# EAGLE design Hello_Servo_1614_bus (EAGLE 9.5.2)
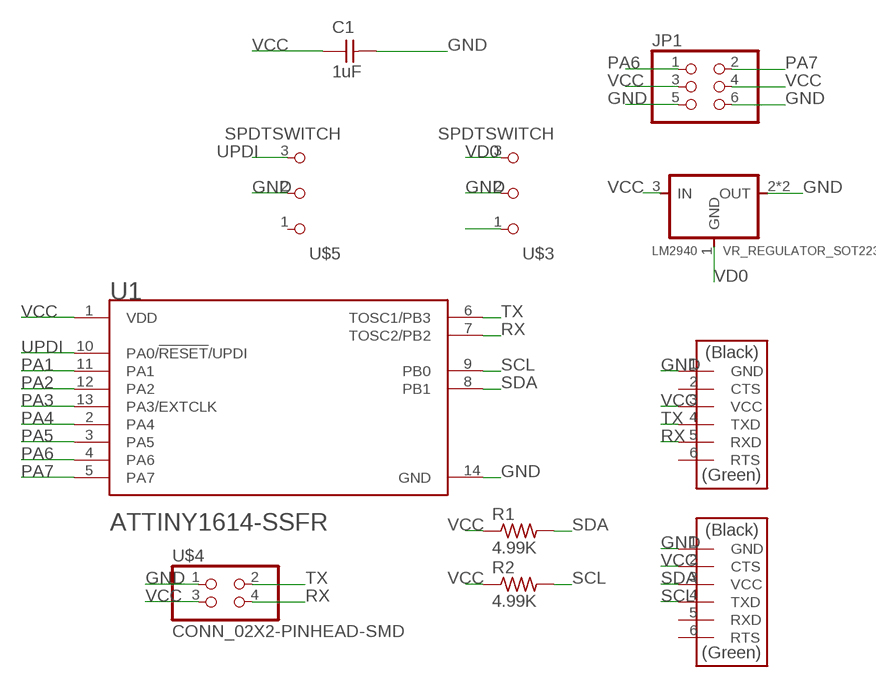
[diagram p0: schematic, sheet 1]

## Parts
C1  1uF  CAP_UNPOLARIZEDFAB  [C1206FAB]
JP1  CONN_03X2-PINHEAD-SMD  [2X03SMD]
LM2940  VR_REGULATOR_SOT223  [SOT223]
R1  4.99K  R1206FAB  [R1206FAB]
R2  4.99K  R1206FAB  [R1206FAB]
U1  MICROCHIP_ATTINY1614-SSFRMICROCHIP_ATTINY1614-SSFR_0_1  [MICROCHIP_ATTINY1614]
U$1  CONN_06_FTDI-SMD-HEADER  [1X06SMD]
U$2  CONN_06_FTDI-SMD-HEADER  [1X06SMD]
U$3  SPDTSWITCH  [SPDTSWITCH]
U$4  CONN_02X2-PINHEAD-SMD  [2X02SMD]
U$5  SPDTSWITCH  [SPDTSWITCH]

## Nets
GND: C1.2 JP1.5 JP1.6 LM2940.2(OUT) LM2940.4(OUT) U1.14(GND) U$1.1(GND) U$2.1(GND) U$3.2 U$4.1 U$5.2
N$2: U$3.1
PA1: U1.11(PA1)
PA2: U1.12(PA2)
PA3: U1.13(PA3/EXTCLK)
PA4: U1.2(PA4)
PA5: U1.3(PA5)
PA6: JP1.1 U1.4(PA6)
PA7: JP1.2 U1.5(PA7)
RX: U1.7(TOSC2/PB2) U$2.5(RXD) U$4.4
SCL: R2.2 U1.9(PB0) U$1.4(TXD)
SDA: R1.2 U1.8(PB1) U$1.3(VCC)
TX: U1.6(TOSC1/PB3) U$2.4(TXD) U$4.2
UPDI: U1.10(PA0/!RESET!/UPDI) U$5.3
VCC [New Class]: C1.1 JP1.3 JP1.4 LM2940.3(IN) R1.1 R2.1 U1.1(VDD) U$1.2(CTS) U$2.3(VCC) U$4.3
VD0: LM2940.1(GND) U$3.3
Unconnected: U$1.5(RXD) U$1.6(RTS) U$2.2(CTS) U$2.6(RTS) U$5.1

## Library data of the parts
C1 = fab:CAP_UNPOLARIZED
JP1 = fab:CONN_03X2-PINHEAD-SMD: PIN HEADER
LM2940 = fab:VR_REGULATOR_SOT223
R1 R2 = fab:R: Resistor (US Symbol)
U1 = Microchip - ATTINY1614-SSFR:MICROCHIP_ATTINY1614-SSFR: IC MCU 8BIT 16KB FLASH 14SOIC; AUTOMOTIVE: No; CENTROID_NOT_SPECIFIED: No; CORE_ARCHITECTURE: AVR; DATASHEET: http://ww1.microchip.com/downloads/en/DeviceDoc/ATtiny1614-DataSheet-DS40001995B.pdf; DATA_BUS_WIDTH: 8bits; DEVICE_CLASS_L1: Integrated Circuits (ICs); DEVICE_CLASS_L2: Embedded Processors and Controllers; DEVICE_CLASS_L3: Microcontrollers; DIGIKEY_DESCRIPTION: IC MCU 8BIT 16KB FLASH 14SOIC; DIGIKEY_PART_NUMBER: ATTINY1614-SSFRCT-ND; FOOTPRINT_PARAMETERS_1: {"fp_type":"SOIC_narrow","params":{"N":{"nom":14,"long name":"Number of leads","min":null,"max":null,"short name":"N","type":"count"},"A":{"nom":false,"long name":"Height","min":false,"max":1750000,"short name":"A","type":"measurement"},"A1":{"nom":false,"long name":"Package clearance","min":100000,"max":250000,"short name":"A1","type":"measurement"},"A2":{"nom":false,"long name":"Package height","min":1250000,"max":false,"short name":"A2","type":"measurement"},"D":{"nom":8650000,"long name":"Package length","min":8550000,"max":8750000,"short name":"D","type":"measurement"},"E":{"nom":6000000,"long name":"Width w/ leads","min":5800000,"max":6200000,"short name":"E","type":"measurement"},"E1":{"nom":3900000,"long name":"Package width","min":3800000,"max":4000000,"short name":"E1","type":"measurement"},"B":{"nom":false,"long name":"Lead width","min":310000,"max":510000,"short name":"B","type":"measurement"},"C":{"nom":false,"long name":"Lead thickness","min":100000,"max":250000,"short name":"C","type":"measurement"},"e":{"nom":1270000,"long name":"Lead pitch","min":null,"max":null,"short name":"e","type":"measurement"},"L":{"nom":false,"long name":"Lead foot length","min":400000,"max":1270000,"short name":"L","type":"measurement"},"PHI":{"nom":false,"long name":"Lead foot angle","min":0,"max":8000000,"short name":"PHI","type":"measurement"},"HT":{"default":"No","long name":"Thermal pad","type":"multichoiceparent","short name":"HT","children":[]},"offset x":{"nom":0,"long name":"X Center offset","min":null,"max":null,"short name":"offset x","type":"measurement"},"offset y":{"nom":0,"long name":"Y Center offset","min":null,"max":null,"short name":"offset y","type":"measurement"},"LS":{"default":"Rounded rectangle","long name":"Land shape","type":"multichoice","short name":"LS"},"LS1":{"default":"Rectangle","long name":"Land shape (Pin 1)","type":"multichoice","short name":"LS1"},"solder toe":{"nom":550000,"long name":"Solder fillet (toe)","min":null,"max":null,"short name":"solder toe","type":"fixedmeasurement"},"solder heel":{"nom":450000,"long name":"Solder fillet (heel)","min":null,"max":null,"short name":"solder heel","type":"fixedmeasurement"},"solder side":{"nom":50000,"long name":"Solder fillet (side)","min":null,"max":null,"short name":"solder side","type":"fixedmeasurement"},"courtyard":{"nom":500000,"long name":"Courtyard","min":null,"max":null,"short name":"courtyard","type":"fixedmeasurement"},"SF":{"default":"A","long name":"Packing level","type":"multichoiceparent","short name":"SF","help":"http://support.upverter.com/customer/portal/articles/978783-what-is-a-footprint-packing-level","children":["solder toe","solder heel","solder side","courtyard"]}}}; FOOTPRINT_PARAMETERS_2: {"fp_type":"SOIC_narrow","params":{"N":{"nom":14,"long name":"Number of leads","min":null,"max":null,"short name":"N","type":"count"},"A":{"nom":false,"long name":"Height","min":false,"max":1750000,"short name":"A","type":"measurement"},"A1":{"nom":false,"long name":"Package clearance","min":100000,"max":250000,"short name":"A1","type":"measurement"},"A2":{"nom":false,"long name":"Package height","min":1250000,"max":false,"short name":"A2","type":"measurement"},"D":{"nom":8650000,"long name":"Package length","min":8550000,"max":8750000,"short name":"D","type":"measurement"},"E":{"nom":6000000,"long name":"Width w/ leads","min":5800000,"max":6200000,"short name":"E","type":"measurement"},"E1":{"nom":3900000,"long name":"Package width","min":3800000,"max":4000000,"short name":"E1","type":"measurement"},"B":{"nom":false,"long name":"Lead width","min":310000,"max":510000,"short name":"B","type":"measurement"},"C":{"nom":false,"long name":"Lead thickness","min":100000,"max":250000,"short name":"C","type":"measurement"},"e":{"nom":1270000,"long name":"Lead pitch","min":null,"max":null,"short name":"e","type":"measurement"},"L":{"nom":false,"long name":"Lead foot length","min":400000,"max":1270000,"short name":"L","type":"measurement"},"PHI":{"nom":false,"long name":"Lead foot angle","min":0,"max":8000000,"short name":"PHI","type":"measurement"},"HT":{"default":"No","long name":"Thermal pad","type":"multichoiceparent","short name":"HT","children":[]},"offset x":{"nom":0,"long name":"X Center offset","min":null,"max":null,"short name":"offset x","type":"measurement"},"offset y":{"nom":0,"long name":"Y Center offset","min":null,"max":null,"short name":"offset y","type":"measurement"},"LS":{"default":"Rounded rectangle","long name":"Land shape","type":"multichoice","short name":"LS"},"LS1":{"default":"Rectangle","long name":"Land shape (Pin 1)","type":"multichoice","short name":"LS1"},"solder toe":{"nom":350000,"long name":"Solder fillet (toe)","min":null,"max":null,"short name":"solder toe","type":"fixedmeasurement"},"solder heel":{"nom":350000,"long name":"Solder fillet (heel)","min":null,"max":null,"short name":"solder heel","type":"fixedmeasurement"},"solder side":{"nom":30000,"long name":"Solder fillet (side)","min":null,"max":null,"short name":"solder side","type":"fixedmeasurement"},"courtyard":{"nom":250000,"long name":"Courtyard","min":null,"max":null,"short name":"courtyard","type":"fixedmeasurement"},"SF":{"default":"B","long name":"Packing level","type":"multichoiceparent","short name":"SF","help":"http://support.upverter.com/customer/portal/articles/978783-what-is-a-footprint-packing-level","children":["solder toe","solder heel","solder side","courtyard"]}}}; FOOTPRINT_PARAMETERS_3: {"fp_type":"SOIC_narrow","params":{"N":{"nom":14,"long name":"Number of leads","min":null,"max":null,"short name":"N","type":"count"},"A":{"nom":false,"long name":"Height","min":false,"max":1750000,"short name":"A","type":"measurement"},"A1":{"nom":false,"long name":"Package clearance","min":100000,"max":250000,"short name":"A1","type":"measurement"},"A2":{"nom":false,"long name":"Package height","min":1250000,"max":false,"short name":"A2","type":"measurement"},"D":{"nom":8650000,"long name":"Package length","min":8550000,"max":8750000,"short name":"D","type":"measurement"},"E":{"nom":6000000,"long name":"Width w/ leads","min":5800000,"max":6200000,"short name":"E","type":"measurement"},"E1":{"nom":3900000,"long name":"Package width","min":3800000,"max":4000000,"short name":"E1","type":"measurement"},"B":{"nom":false,"long name":"Lead width","min":310000,"max":510000,"short name":"B","type":"measurement"},"C":{"nom":false,"long name":"Lead thickness","min":100000,"max":250000,"short name":"C","type":"measurement"},"e":{"nom":1270000,"long name":"Lead pitch","min":null,"max":null,"short name":"e","type":"measurement"},"L":{"nom":false,"long name":"Lead foot length","min":400000,"max":1270000,"short name":"L","type":"measurement"},"PHI":{"nom":false,"long name":"Lead foot angle","min":0,"max":8000000,"short name":"PHI","type":"measurement"},"HT":{"default":"No","long name":"Thermal pad","type":"multichoiceparent","short name":"HT","children":[]},"offset x":{"nom":0,"long name":"X Center offset","min":null,"max":null,"short name":"offset x","type":"measurement"},"offset y":{"nom":0,"long name":"Y Center offset","min":null,"max":null,"short name":"offset y","type":"measurement"},"LS":{"default":"Rounded rectangle","long name":"Land shape","type":"multichoice","short name":"LS"},"LS1":{"default":"Rectangle","long name":"Land shape (Pin 1)","type":"multichoice","short name":"LS1"},"solder toe":{"nom":150000,"long name":"Solder fillet (toe)","min":null,"max":null,"short name":"solder toe","type":"fixedmeasurement"},"solder heel":{"nom":250000,"long name":"Solder fillet (heel)","min":null,"max":null,"short name":"solder heel","type":"fixedmeasurement"},"solder side":{"nom":10000,"long name":"Solder fillet (side)","min":null,"max":null,"short name":"solder side","type":"fixedmeasurement"},"courtyard":{"nom":100000,"long name":"Courtyard","min":null,"max":null,"short name":"courtyard","type":"fixedmeasurement"},"SF":{"default":"C","long name":"Packing level","type":"multichoiceparent","short name":"SF","help":"http://support.upverter.com/customer/portal/articles/978783-what-is-a-footprint-packing-level","children":["solder toe","solder heel","solder side","courtyard"]}}}; FOOTPRINT_VARIANT_NAME_0: Recommended_Land_Pattern; FOOTPRINT_VARIANT_NAME_1: IPC_A; FOOTPRINT_VARIANT_NAME_2: IPC_B; FOOTPRINT_VARIANT_NAME_3: IPC_C; FREQUENCY: 16MHz; HEIGHT: 1.75mm; INTERFACE: I2C,SPI,UART,USART,2-Wire,LIN,IrDA; IPC_LAND_PATTERN_NAME: SOIC127P600X175-14; LEAD_FREE: Yes; MAX_SUPPLY_VOLTAGE: 5.5V; MEMORY_SIZE: 16KBytes; MEMORY_TYPE: FLASH; MF: Microchip; MFG_PACKAGE_IDENT: C04-065-D3X; MFG_PACKAGE_IDENT_DATE: 0; MFG_PACKAGE_IDENT_REV: D; MIN_SUPPLY_VOLTAGE: 1.8V; MOUSER_DESCRIPTION: 8-Bit AVR Microcontroller 16Kbyte Flash 2Kbyte SRAM 14-Pin SOIC T/R; MOUSER_PART_NUMBER: 556-ATTINY1614SSFR; MPN: ATTINY1614-SSFR; NOMINAL_SUPPLY_CURRENT: 2.6-10200uA; NUMBER_OF_A/D_CONVERTERS: 2; NUMBER_OF_ADC_CHANNELS: 14; NUMBER_OF_CORES: 1; NUMBER_OF_I/OS: 12; NUMBER_OF_I2C_CHANNELS: 1; NUMBER_OF_PWM_CHANNELS: 1; NUMBER_OF_SPI_CHANNELS: 1; NUMBER_OF_TIMERS/COUNTERS: 5; NUMBER_OF_UART_CHANNELS: 1; PACKAGE: SOIC14; PREFIX: U; RAM_SIZE: 2KBytes; ROHS: Yes; STANDOFF_HEIGHT: 0.1mm; TEMPERATURE_RANGE_HIGH: +125°C; TEMPERATURE_RANGE_LOW: -40°C; VERIFICATION_VERSION: 0.0.0.3
U$1 U$2 = fab:CONN_06_FTDI-SMD-HEADER
U$3 U$5 = fab:SPDTSWITCH
U$4 = fab:CONN_02X2-PINHEAD-SMD

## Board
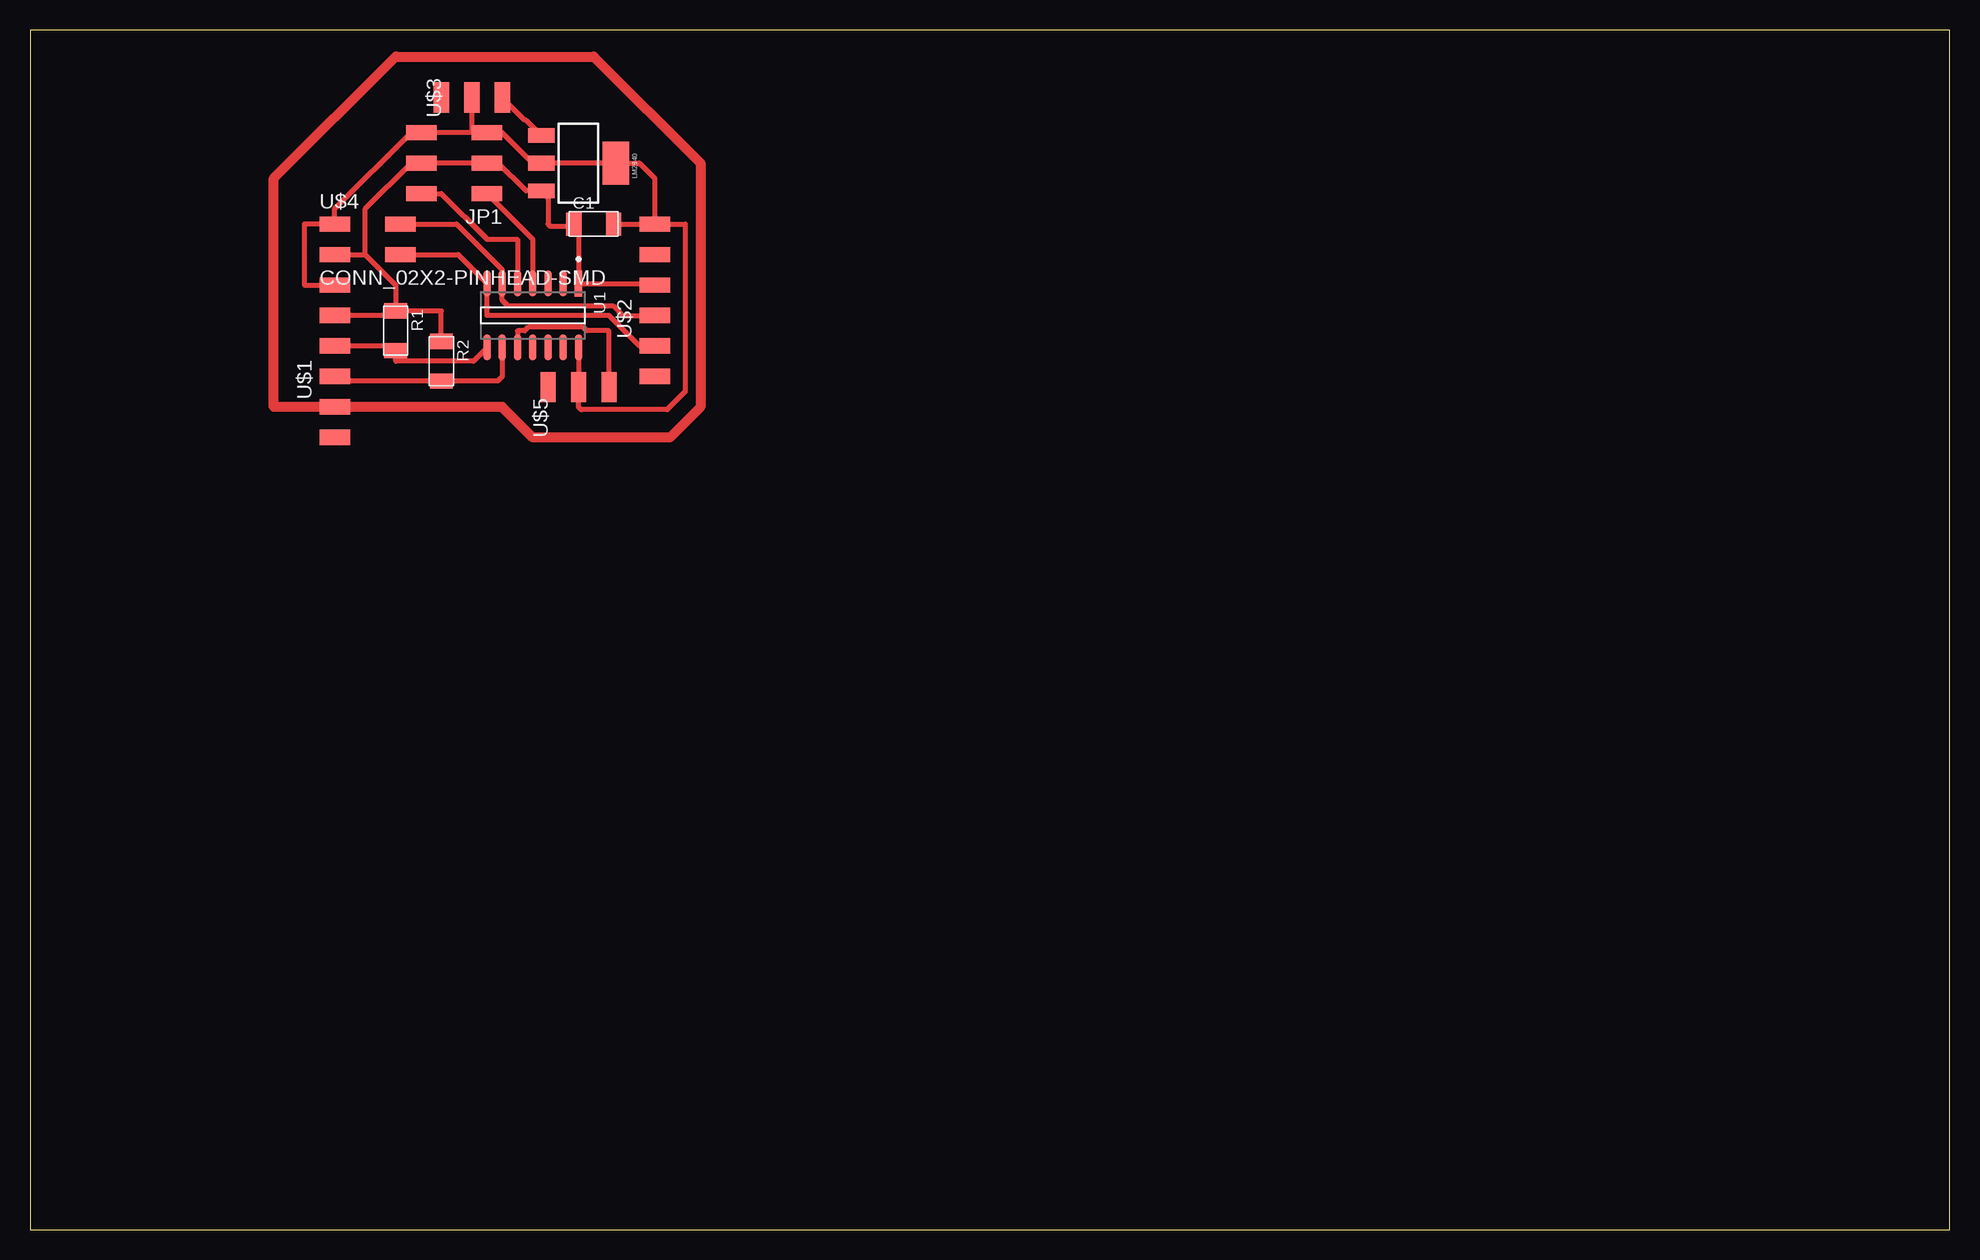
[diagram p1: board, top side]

Size 160 x 100 mm. Coordinates in mm from the lower left corner, seen from the top.
Outline: 0,0 160,0 160,100 0,100 0,0
Copper layers (1*16): Top 0.035mm / dielectric 1.5mm / Bottom 0.035mm
Design rules "default *": minimum track width 16mil, minimum drill 0.35mm, track to track 16mil, track to pad 16mil, pad to pad 16mil, via to via 16mil, smd to smd 6mil, copper to edge 40mil, drill to drill 6mil, minimum pad ring 10mil, minimum via ring 8mil, stop-mask expansion 4mil, vias tented up to drill 0mil, thermal gap 10mil

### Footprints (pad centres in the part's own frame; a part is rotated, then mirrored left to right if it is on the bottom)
C1206FAB = smd 1.27 x 1.905: 1 -1.651,0; 2 1.651,0
2X03SMD = smd 2.54 x 1.27: 1 -2.54,2.54; 2 2.92,2.54; 3 -2.54,0; 4 2.92,0; 5 -2.54,-2.54; 6 2.92,-2.54
SOT223 = smd 1.219 x 2.235: 1 -2.311,-3.099; 2 0,-3.099; 3 2.311,-3.099 | smd 3.6 x 2.2: 4 0,3.099
R1206FAB = smd 1.27 x 1.905: 1 -1.651,0; 2 1.651,0
MICROCHIP_ATTINY1614 = smd 2.169 x 0.622: 1 -2.67,3.81; 2 -2.67,2.54; 3 -2.67,1.27; 4 -2.67,0; 5 -2.67,-1.27; 6 -2.67,-2.54; 7 -2.67,-3.81; 8 2.67,-3.81; 9 2.67,-2.54; 10 2.67,-1.27; 11 2.67,0; 12 2.67,1.27; 13 2.67,2.54; 14 2.67,3.81
1X06SMD = smd 2.54 x 1.27: 1 0,6.35; 2 0,3.81; 3 0,1.27; 4 0,-1.27; 5 0,-3.81; 6 0,-6.35
SPDTSWITCH = smd 2.54 x 1.27: 1 0.38,2.54; 2 0.38,0; 3 0.38,-2.54
2X02SMD = smd 2.54 x 1.27: 1 -2.54,1.27; 2 2.92,1.27; 3 -2.54,-1.27; 4 2.92,-1.27

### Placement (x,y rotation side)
C1  46.99,83.82 0 top
JP1  35.56,88.9 180 top
LM2940  45.72,88.9 270 top
R1  30.48,74.93 270 top
R2  34.29,72.39 270 top
U1  41.91,76.2 270 top
U$1  25.4,72.39 0 top
U$2  52.07,77.47 0 top
U$3  36.83,93.98 90 top
U$4  27.94,82.55 0 top
U$5  45.72,69.85 90 top

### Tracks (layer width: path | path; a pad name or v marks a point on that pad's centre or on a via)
GND
  Top 0.406: C1.2 U$2.1 | U1.14 U$5.2 45.72,68.58 45.95,68.35 53.11,68.35 54.61,69.85 54.61,83.82 U$2.1 | U$3.2 36.83,91.44 JP1.5 | U$2.1 52.07,87.63 50.8,88.9 LM2940.4 LM2940.2 41.91,88.9 39.37,91.44 JP1.5 | JP1.5 JP1.6 31.75,91.44 25.4,85.09 U$4.1 22.86,83.82 22.86,78.74 U$1.1
N$1
  Top 0.813: 30.48,97.79 46.99,97.79 55.88,88.9 55.88,68.58 53.34,66.04 41.91,66.04 39.37,68.58 20.32,68.58 20.32,87.63 30.48,97.79
PA6
  Top 0.406: JP1.1 41.91,82.55 U1.4
PA7
  Top 0.406: JP1.2 34.29,86.36 38.1,82.55 40.64,82.55 U1.5
RX
  Top 0.406: U$2.5 50.8,73.66 48.26,76.2 38.1,76.2 U1.7 35.69,81.28 U$4.4
SCL
  Top 0.406: U1.9 39.37,71.12 38.99,70.74 R2.2 25.78,70.74 U$1.4
SDA
  Top 0.406: U1.8 36.96,72.39 30.48,72.39 R1.2 30.1,73.66 U$1.3
TX
  Top 0.406: U$2.4 49.41,76.2 48.6,77.01 39.83,77.01 39.37,77.47 39.37,78.74 U1.6 39.37,80.01 35.56,83.82 U$4.2
UPDI
  Top 0.406: U$5.3 48.26,74.93 46.4,74.93 46.1,75.22 41.53,75.22 41.23,74.93 40.64,74.93 U1.10
VCC
  Top 0.406: C1.1 45.53,83.63 | 45.53,83.63 45.72,83.44 U1.1 51.94,78.87 U$2.3 | 45.53,83.63 43.37,83.63 43.18,83.82 43.18,86.03 LM2940.3 41.35,86.59 39.04,88.9 JP1.3 JP1.4 31.75,88.9 27.94,85.09 27.94,81.28 | R2.1 34.29,76.58 R1.1 | R1.1 30.1,76.2 U$1.2 | 27.94,81.28 30.48,78.74 R1.1 | U$4.3 27.94,81.28
VD0
  Top 0.406: U$3.3 41.25,92.48 41.35,92.48 LM2940.1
